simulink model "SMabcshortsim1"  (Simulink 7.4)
settings: Solver=ode45  StartTime=0.0  StopTime=10  MaxStep=2e-4  RelTol=1e-3
InitFcn:
  | smparamshortsim1
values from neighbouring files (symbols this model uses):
  Bm = 0.10    (= 0.1)    [IMabc2.m]    (also in imabcparam.m = 0.01; IMabcrun0.m = 0.01; IMabcrun1.m = 0.001; IMcur0.m = 1e-06)
  D = str2num(get(h,'string'))    [acttrcalc1.m]
  gam = 2*pi/3    (= 2.09439510239)    [IMabc2.m]    (also in IMabcf0.m; IMabcf1.m; imabcparam.m; IMabcrun0.m)
  H = 0.60    (= 0.6)    [IMabc2.m]    (also in IMcur0.m = 0.3; imdef0vec.m = 0.3; imdef1vec.m = 0.3; imdef2vec.m = 0.3)
  Lm = eval(get(hLm,'String'))    [im3d.m]    (also in IMabc2.m = 4.5; imabcparam.m = 0.0847; IMabcrun0.m = 0.0847; IMabcrun1.m = 0.0847)
  Lrr = [Lr   -Lm/2 -Lm/2    [IMabc2.m]    (also in IMabcf0.m = [Lr   -Lm1/2 -Lm1/2; IMabcf1.m = [Lr   -Lm1/2 -Lm1/2)
  Lss = [Ls   -Lm/2 -Lm/2    [IMabc2.m]    (also in IMabcf0.m = [Ls   -Lm1/2 -Lm1/2; IMabcf1.m = [Ls   -Lm1/2 -Lm1/2)
  R = str2num(get(h,'string'))    [acttrcalc1.m]    (also in IMabc2.m = diag([Rs Rs Rs Rr Rr Rr]); IMabcf0.m = diag([Rs Rs Rs Rr Rr Rr]); IMabcf1.m = diag([Rs Rs Rs Rr Rr Rr]); IMcurf0.m = diag([Rs Rs Rr Rr]))
  Vs = abs(Vas)    [calc0.m]    (also in Ccurverun.m = 1; IMabc2.m = 1; IMabcrun0.m = Vll*sqrt(2/3); IMabcrun1.m = Vll*sqrt(2/3))
  wo = 2*pi*freq0    [calc0.m]    (also in IMabc2.m = 376.991118431; imabcparam.m = 376.991118431; IMabcrun0.m = 376.991118431; IMabcrun1.m = 376.991118431)
undefined symbols (not defined in the file or in its folder): Laf, Lakd, Lakq, phas, Rf, Row, vector

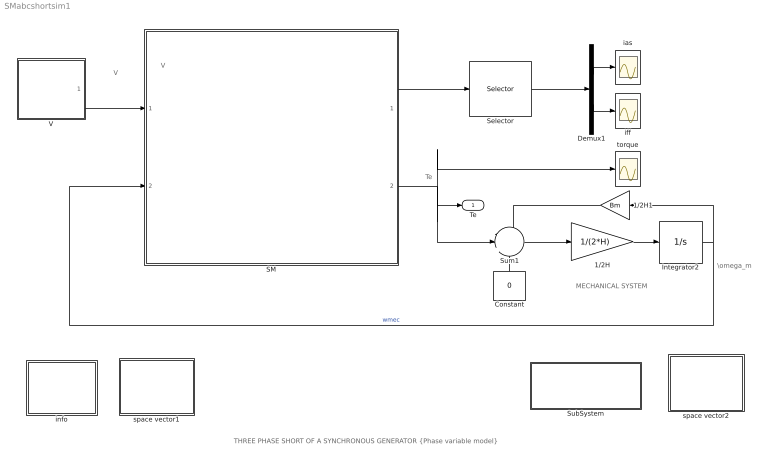
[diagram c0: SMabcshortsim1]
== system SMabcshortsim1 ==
  note: MECHANICAL SYSTEM
  note: Te
  note: \omega_m
  note: V
  note: I
  note: V
  note: THREE PHASE SHORT OF A SYNCHRONOUS GENERATOR {Phase variable model}
  1/2H : Gain  Gain=1/(2*H)  ParameterDataType=sfix(16)  ParameterScaling=2^0  OutDataType=sfix(16)  OutScaling=2^0
  1/2H1 : Gain  Gain=Bm  ParameterDataType=sfix(16)  ParameterScaling=2^0  OutDataType=sfix(16)  OutScaling=2^0
  Constant : Constant  Value=0  OutDataType=sfix(16)  OutScaling=2^0
  Demux1 : Demux  Outputs=2
  Integrator2 : Integrator  InitialCondition=1
  SM : Subsystem
  Selector : Selector  InputPortWidth=6  IndexOptions=Index vector (dialog)  Indices=[1 4 ]  OutputSizes=1
  SubSystem : Subsystem
  Sum1 : Sum  Inputs=-|+|-  OutDataType=sfix(16)  OutScaling=2^0
  V : Subsystem
  ias : Scope
  iff : Scope
  info : Subsystem
  space vector1 : Subsystem
  space vector2 : Subsystem
  torque : Scope
  Te : Outport
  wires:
  1/2H/1 -> Integrator2/1
  Integrator2/1 -> 1/2H1/1, SM/2(wm)  "wmec"
  V/1(V) -> SM/1(V)
  Sum1/1 -> 1/2H/1
  Demux1/2 -> iff/1
  Demux1/1 -> ias/1
  1/2H1/1 -> Sum1/1
  SM/1(I) -> Selector/1
  SM/2(Te) -> Sum1/2, torque/1, Te/1
  Constant/1 -> Sum1/3
  Selector/1 -> Demux1/1

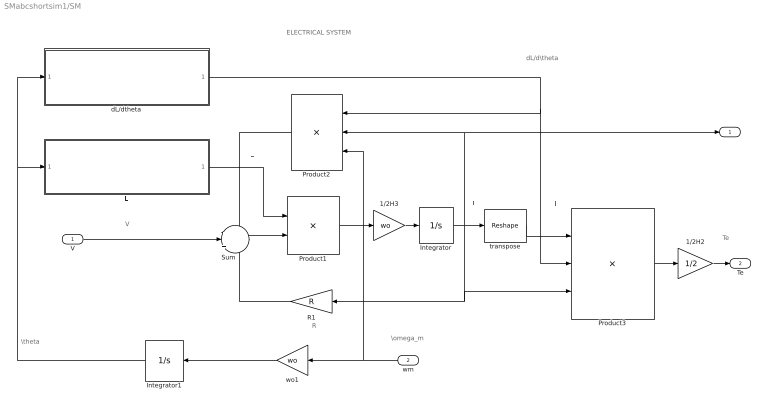
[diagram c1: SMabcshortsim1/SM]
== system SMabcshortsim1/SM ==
  note: \theta
  note: dL/d\theta
  note: L
  note: V
  note: ELECTRICAL SYSTEM
  note: I'
  note: I
  note: Te
  note: I
  note: \omega_m
  note: R
  V : Inport  OutDataType=sfix(16)  OutScaling=2^0
  wm : Inport  Port=2  OutDataType=sfix(16)  OutScaling=2^0
  1/2H2 : Gain  Gain=1/2  ParameterDataType=sfix(16)  ParameterScaling=2^0  OutDataType=sfix(16)  OutScaling=2^0
  1/2H3 : Gain  Gain=wo  ParameterDataType=sfix(16)  ParameterScaling=2^0  OutDataType=sfix(16)  OutScaling=2^0
  Integrator : Integrator  InitialCondition=[0 ;0 ;0; Vs/Lm;0 ;0 ]  ZeroCross=off
  Integrator1 : Integrator  InitialCondition=phas
  L : Subsystem
  Product1 : Product  Inputs=/*  Multiplication=Matrix(*)  OutDataType=sfix(16)  OutScaling=2^0
  Product2 : Product  Inputs=***  Multiplication=Matrix(*)  OutDataType=sfix(16)  OutScaling=2^0
  Product3 : Product  Inputs=3  Multiplication=Matrix(*)  OutDataType=sfix(16)  OutScaling=2^0
  R1 : Gain  Gain=R  Multiplication=Matrix(K*u)  ParameterDataType=sfix(16)  ParameterScaling=2^0  OutDataType=sfix(16)  OutScaling=2^0
  Sum : Sum  Inputs=-|+|-  OutDataType=sfix(16)  OutScaling=2^0
  dL/dtheta : Subsystem
  transpose : Reshape  OutputDimensionality=Row vector (2-D)  OutputDimensions=[1,6]
  wo1 : Gain  Gain=wo  ParameterDataType=sfix(16)  ParameterScaling=2^0  OutDataType=sfix(16)  OutScaling=2^0
  I : Outport
  Te : Outport  Port=2
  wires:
  wo1/1 -> Integrator1/1
  R1/1 -> Sum/3
  1/2H3/1 -> Integrator/1
  Integrator/1 -> transpose/1, Product2/2, I/1, R1/1, Product3/3
  L/1(L) -> Product1/1
  Integrator1/1 -> dL/dtheta/1(theta1), L/1(theta)
  Product3/1 -> 1/2H2/1
  dL/dtheta/1(dLdtheta) -> Product2/1, Product3/2
  Product2/1 -> Sum/1
  transpose/1 -> Product3/1
  Sum/1 -> Product1/2
  Product1/1 -> 1/2H3/1
  wm/1 -> Product2/3, wo1/1
  V/1 -> Sum/2
  1/2H2/1 -> Te/1

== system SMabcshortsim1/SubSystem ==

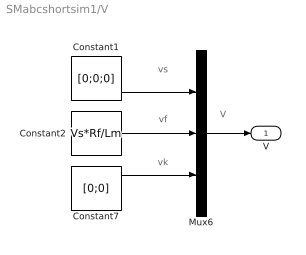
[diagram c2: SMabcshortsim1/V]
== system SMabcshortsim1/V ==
  note: vk
  note: vs
  note: vf
  note: V
  Constant1 : Constant  Value=[0;0;0]  VectorParams1D=off  OutDataType=sfix(16)  OutScaling=2^0
  Constant2 : Constant  Value=Vs*Rf/Lm  VectorParams1D=off  OutDataType=sfix(16)  OutScaling=2^0
  Constant7 : Constant  Value=[0;0]  VectorParams1D=off  OutDataType=sfix(16)  OutScaling=2^0
  Mux6 : Mux  Inputs=3
  V : Outport
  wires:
  Constant7/1 -> Mux6/3
  Constant2/1 -> Mux6/2
  Constant1/1 -> Mux6/1
  Mux6/1 -> V/1

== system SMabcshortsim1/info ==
  note: A cylindrical rotor synchronous generator is running under open circuit conditions when a three-phase fault is placed at the stator terminals. The dynamic equations are expressed in matrix form in terms the phase variables, namely the stator currents ias, ibs, ics; the rotor field current iff; the d-axis and q-axis damper currents idk and iqk; the angular speed wm; and the displacement angle theta between stator as-axis and rotor direct axis. Torque and current responses are plotted. A Matlab script file for the identical system operation is given in the file >.
  note: THREE-PHASE SHORT OF A SYNCHRONOUS GENERATOR (Phase variable model) [pu]

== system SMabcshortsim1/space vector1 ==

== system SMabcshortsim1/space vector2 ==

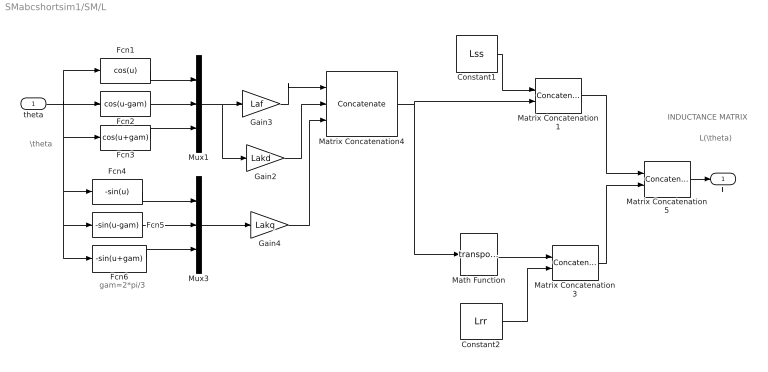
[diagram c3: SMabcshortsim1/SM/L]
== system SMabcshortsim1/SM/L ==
  note: INDUCTANCE MATRIX
  note: gam=2*pi/3
  note: \theta
  note: L(\theta)
  theta : Inport  OutDataType=sfix(16)  OutScaling=2^0
  Constant1 : Constant  Value=Lss  VectorParams1D=off  OutDataType=sfix(16)  OutScaling=2^0
  Constant2 : Constant  Value=Lrr  VectorParams1D=off  OutDataType=sfix(16)  OutScaling=2^0
  Fcn1 : Fcn  Expr=cos(u)
  Fcn2 : Fcn  Expr=cos(u-gam)
  Fcn3 : Fcn  Expr=cos(u+gam)
  Fcn4 : Fcn  Expr=-sin(u)
  Fcn5 : Fcn  Expr=-sin(u-gam)
  Fcn6 : Fcn  Expr=-sin(u+gam)
  Gain2 : Gain  Gain=Lakd  ParameterDataType=sfix(16)  ParameterScaling=2^0  OutDataType=sfix(16)  OutScaling=2^0
  Gain3 : Gain  Gain=Laf  ParameterDataType=sfix(16)  ParameterScaling=2^0  OutDataType=sfix(16)  OutScaling=2^0
  Gain4 : Gain  Gain=Lakq  ParameterDataType=sfix(16)  ParameterScaling=2^0  OutDataType=sfix(16)  OutScaling=2^0
  Math Function : Math  Operator=transpose
  Matrix Concatenation1 : Concatenate  Mode=Multidimensional array  ConcatenateDimension=2
  Matrix Concatenation3 : Concatenate  Mode=Multidimensional array  ConcatenateDimension=2
  Matrix Concatenation4 : Concatenate  NumInputs=3  Mode=Multidimensional array  ConcatenateDimension=2
  Matrix Concatenation5 : Concatenate  Mode=Multidimensional array
  Mux1 : Mux  Inputs=3
  Mux3 : Mux  Inputs=3
  L : Outport
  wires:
  Matrix Concatenation5/1 -> L/1
  Matrix Concatenation4/1 -> Matrix Concatenation1/2, Math Function/1
  Mux1/1 -> Gain3/1, Gain2/1
  Matrix Concatenation1/1 -> Matrix Concatenation5/1
  Constant1/1 -> Matrix Concatenation1/1
  Fcn3/1 -> Mux1/3
  Fcn2/1 -> Mux1/2
  Fcn1/1 -> Mux1/1
  theta/1 -> Fcn2/1, Fcn1/1, Fcn3/1, Fcn6/1, Fcn5/1, Fcn4/1
  Gain3/1 -> Matrix Concatenation4/1
  Gain2/1 -> Matrix Concatenation4/2
  Fcn5/1 -> Mux3/2
  Fcn4/1 -> Mux3/1
  Fcn6/1 -> Mux3/3
  Mux3/1 -> Gain4/1
  Gain4/1 -> Matrix Concatenation4/3
  Math Function/1 -> Matrix Concatenation3/1
  Constant2/1 -> Matrix Concatenation3/2
  Matrix Concatenation3/1 -> Matrix Concatenation5/2

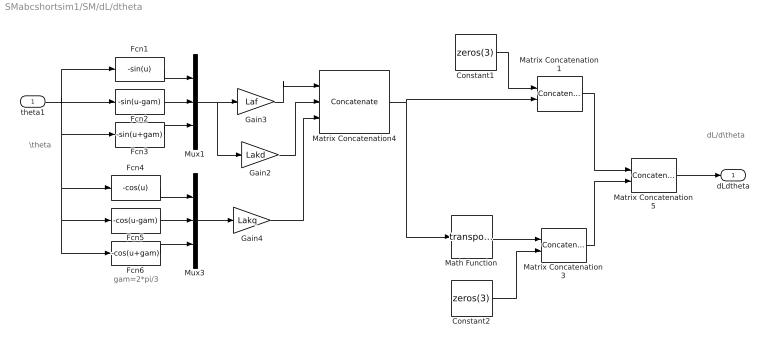
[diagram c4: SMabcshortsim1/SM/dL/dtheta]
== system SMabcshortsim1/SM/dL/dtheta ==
  note: dL/d\theta
  note: gam=2*pi/3
  note: \theta
  theta1 : Inport  OutDataType=sfix(16)  OutScaling=2^0
  Constant1 : Constant  Value=zeros(3)  VectorParams1D=off  OutDataType=sfix(16)  OutScaling=2^0
  Constant2 : Constant  Value=zeros(3)  VectorParams1D=off  OutDataType=sfix(16)  OutScaling=2^0
  Fcn1 : Fcn  Expr=-sin(u)
  Fcn2 : Fcn  Expr=-sin(u-gam)
  Fcn3 : Fcn  Expr=-sin(u+gam)
  Fcn4 : Fcn  Expr=-cos(u)
  Fcn5 : Fcn  Expr=-cos(u-gam)
  Fcn6 : Fcn  Expr=-cos(u+gam)
  Gain2 : Gain  Gain=Lakd  ParameterDataType=sfix(16)  ParameterScaling=2^0  OutDataType=sfix(16)  OutScaling=2^0
  Gain3 : Gain  Gain=Laf  ParameterDataType=sfix(16)  ParameterScaling=2^0  OutDataType=sfix(16)  OutScaling=2^0
  Gain4 : Gain  Gain=Lakq  ParameterDataType=sfix(16)  ParameterScaling=2^0  OutDataType=sfix(16)  OutScaling=2^0
  Math Function : Math  Operator=transpose
  Matrix Concatenation1 : Concatenate  Mode=Multidimensional array  ConcatenateDimension=2
  Matrix Concatenation3 : Concatenate  Mode=Multidimensional array  ConcatenateDimension=2
  Matrix Concatenation4 : Concatenate  NumInputs=3  Mode=Multidimensional array  ConcatenateDimension=2
  Matrix Concatenation5 : Concatenate  Mode=Multidimensional array
  Mux1 : Mux  Inputs=3
  Mux3 : Mux  Inputs=3
  dLdtheta : Outport
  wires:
  Matrix Concatenation5/1 -> dLdtheta/1
  Matrix Concatenation4/1 -> Matrix Concatenation1/2, Math Function/1
  Mux1/1 -> Gain3/1, Gain2/1
  Matrix Concatenation1/1 -> Matrix Concatenation5/1
  Constant1/1 -> Matrix Concatenation1/1
  Fcn3/1 -> Mux1/3
  Fcn2/1 -> Mux1/2
  Fcn1/1 -> Mux1/1
  theta1/1 -> Fcn2/1, Fcn1/1, Fcn3/1, Fcn6/1, Fcn5/1, Fcn4/1
  Gain3/1 -> Matrix Concatenation4/1
  Gain2/1 -> Matrix Concatenation4/2
  Fcn5/1 -> Mux3/2
  Fcn4/1 -> Mux3/1
  Fcn6/1 -> Mux3/3
  Mux3/1 -> Gain4/1
  Gain4/1 -> Matrix Concatenation4/3
  Math Function/1 -> Matrix Concatenation3/1
  Constant2/1 -> Matrix Concatenation3/2
  Matrix Concatenation3/1 -> Matrix Concatenation5/2
